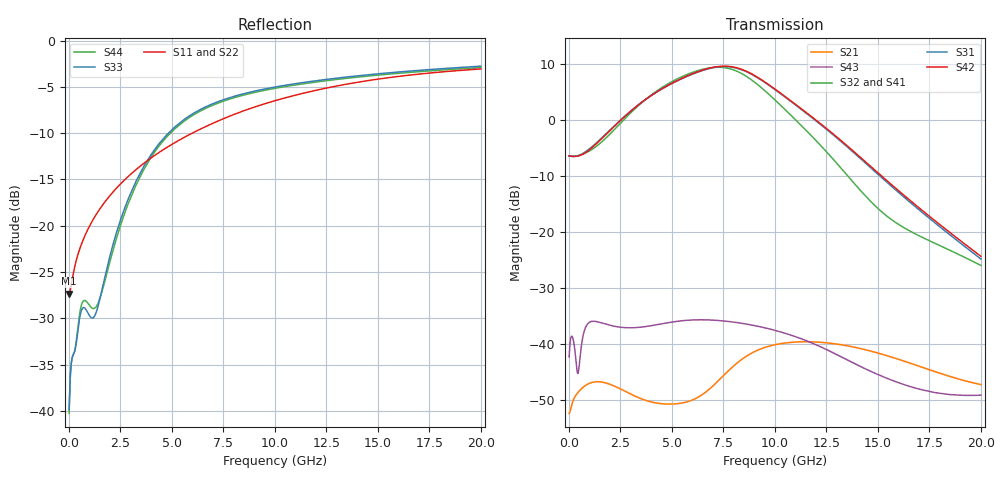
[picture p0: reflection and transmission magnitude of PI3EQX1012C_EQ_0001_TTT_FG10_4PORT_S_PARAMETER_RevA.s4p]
! NPort=4 DATA=2000 NOISE=0 GROUPDELAY=0 COMPLEX_DATAFORMAT=POLAR
! NumOfBlock=1 NumOfParam=0
! .MODEL Smodel S TSTONEFILE=PI3EQX1012C_EQ_0001_TTT_FG10_4PORT_S_PARAMETER_RevA.s4p TYPE=S
!  -- The above .MODEL line can be used for the S element in the netlist.
! The s parameter is extracted from the linear redriver, it is not bi-directional; only s(4,1)s(4,2) and s(3,1)s(3,2)
! should be the insertion loss
!Port definition:
!Port1 = input+
!Port2 = input-
!Port3 = output+
!Port4 = output-
# Hz S MA R  50
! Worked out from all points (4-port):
!   2000 points, 10 MHz to 20 GHz, reference 50 ohm
!   strongest paths, dB at 10 MHz, 5.01 GHz, 10.01 GHz, 15.01 GHz, 20 GHz:
!     S42: -6.4, 6.6, 5.5, -9.4, -24.4
!     S31: -6.4, 6.6, 5.4, -9.7, -24.8
!     S32: -6.4, 6.9, 3.6, -15.8, -26.0
!     S41: -6.4, 6.9, 3.7, -16.0, -26.3
!     S43: -42.4, -36.1, -37.6, -45.5, -49.2
!     S21: -52.4, -50.8, -40.2, -41.7, -47.3
!   lowest |S11| = -27.3 dB at 10 MHz (marker M1), VSWR 1.09, Z = 45.9 - j0.123 ohm
!   |S11| at or under -10 dB: start of sweep to 5.988 GHz
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1e7  0.04301 -178.2  0.002379 1.5  0.0008102 -0.5  0.0008039 -0.5
     0.002388 1.5  0.04109 -178.1  0.000927 -0.5  0.0009197 -0.5
     0.4783 -0.3  0.4774 179.8  0.01016 -4.0  0.007598 -25.7
     0.4769 179.8  0.4792 -0.3  0.007615 -25.8  0.009722 -4.1
5.19e9  0.2831 -123.9  0.002938 14.8  0.000304 -58.9  0.000303 -59.6
        0.002903 14.3  0.2878 -123.1  0.0003451 -59.7  0.0003439 -60.5
        2.216 -110.8  2.307 83.7  0.3452 -94.3  0.01564 18.2
        2.307 84.1  2.226 -108.9  0.01582 15.0  0.3374 -94.0
7.11e9  0.3625 -124.7  0.004568 40.4  0.0002377 -55.8  0.0002356 -57.2
        0.004401 40.5  0.3681 -124.2  0.000268 -57.0  0.0002657 -58.4
        2.968 165.2  2.969 -0.7  0.4618 -109.9  0.01663 -11.6
        2.99 -0.9  2.992 167.4  0.01622 -13.0  0.4536 -109.8
8.39e9  0.4138 -126.2  0.007447 33.6  0.000221 -54.1  0.0002178 -55.6
        0.007247 34.7  0.42 -125.7  0.0002475 -55.3  0.000244 -56.8
        2.82 100.6  2.608 -64.3  0.513 -117.3  0.01562 -28.9
        2.636 -65.0  2.847 103.1  0.01525 -29.6  0.5045 -117.2
9.96e9  0.4718 -128.6  0.009901 10.6  0.0002109 -54.1  0.0002066 -55.7
        0.009762 11.7  0.4788 -128.2  0.0002343 -55.2  0.0002298 -56.7
        1.901 28.7  1.543 -132.5  0.5598 -124.0  0.01358 -47.2
        1.563 -133.8  1.922 31.5  0.01325 -47.8  0.5509 -123.9
1.223e10  0.5459 -132.4  0.01038 -19.5  0.0002001 -57.5  0.0001949 -59.0
          0.0103 -18.8  0.5544 -132.0  0.000221 -58.1  0.0002156 -59.7
          0.9096 -55.0  0.591 154.4  0.6115 -130.7  0.009665 -68.4
          0.5952 151.9  0.9249 -51.5  0.009368 -69.0  0.6018 -130.6
2e10  0.7027 -144.5  0.004332 -59.5  0.0001467 -72.3  0.0001416 -73.8
      0.004316 -58.4  0.7176 -144.3  0.0001627 -72.1  0.000157 -73.7
      0.05731 111.6  0.05021 39.1  0.7272 -143.5  0.003552 -51.6
      0.04852 37.1  0.06055 116.3  0.003471 -48.9  0.7152 -143.3
